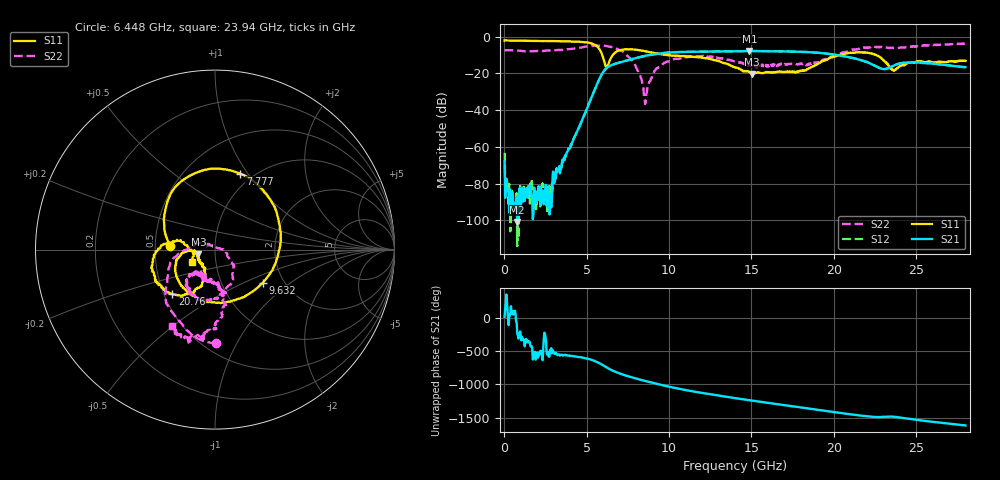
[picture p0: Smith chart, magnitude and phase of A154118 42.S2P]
!  2-Port S-parameters saved by WinCal
! VAR MeasName=S-Parameters (CALIBRATED_DATA) read from VNA (N5230A)
! VAR MeasDate=2015-9-10 14:37:42
! VAR NAME=A154118 42
! VAR FILENAME=A154118 42.S2P
! VAR DATE=2015-9-10 14:37:42
! VAR PHYS_PORTS=1,2
# Hz S DB R 50
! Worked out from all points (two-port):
!   801 points, 10 MHz to 28 GHz, reference 50 ohm
!   highest |S21| = -7.89 dB at 14.88 GHz (marker M1); lowest = -101.0 dB at 779.7 MHz (marker M2)
!   |S21| within 3 dB of the highest: 8.387 GHz to 20.75 GHz (12.37 GHz wide, 84.9 % of centre)
!   lowest |S11| = -20.3 dB at 15.05 GHz (marker M3), VSWR 1.21, Z = 41.5 - j2.24 ohm
!   |S11| at or under -10 dB: 5.938 GHz to 6.588 GHz (650.3 MHz wide, 10.4 % of centre); 9.806 GHz to 20.41 GHz (10.6 GHz wide, 70.2 % of centre); 22.58 GHz to end of sweep
!   |S22| runs from -36.7 to -3.7 dB; largest |S21 - S12| = 0.007
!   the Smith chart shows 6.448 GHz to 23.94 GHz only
!   S11 on the Smith chart (normalised r, x): 6.448 GHz: 0.60, +0.03; 7.777 GHz: 0.88, +0.92; 9.632 GHz: 1.57, -0.64; 20.76 GHz: 0.55, -0.31; 23.94 GHz: 0.76, -0.11
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1e7  -2.16 179.7  -67.96 19.1  -63.22 24.7  -7.49 179.8
1.849375e8  -2.16 177.2  -82.53 135.5  -82.31 15.3  -7.43 174.3
7.79725e8  -2.28 169.3  -100.98 121.6  -114.08 176.7  -7.60 155.9
2.774012e9  -2.49 142.1  -91.00 -118.1  -93.91 86.2  -7.66 97.4
4.698325e9  -3.00 98.2  -45.83 127.2  -45.63 127.0  -5.93 12.7
5.712962e9  -6.21 31.1  -24.14 47.7  -24.12 47.5  -4.94 -43.2
6.1678e9  -16.44 -82.5  -17.44 -17.7  -17.43 -17.8  -5.12 -71.3
6.4477e9  -11.97 175.2  -15.75 -56.6  -15.73 -57.0  -5.65 -89.4
7.777225e9  -7.02 71.4  -12.23 -175.4  -12.23 -175.5  -13.22 -170.3
8.54695e9  -7.97 30.1  -10.55 132.8  -10.53 132.9  -36.74 81.1
9.351662e9  -9.36 -17.8  -9.37 83.2  -9.31 83.0  -17.00 -43.3
9.631562e9  -9.79 -34.5  -9.04 67.1  -9.01 66.9  -14.90 -56.5
1.131096e10  -10.88 -118.1  -8.33 -17.7  -8.31 -18.4  -11.09 -95.9
1.4005e10  -16.74 -179.2  -8.02 -124.9  -8.02 -125.3  -13.55 -134.4
1.487969e10  -19.38 -168.9  -7.89 -156.6  -7.88 -157.3  -15.51 -127.0
1.505462e10  -20.33 -163.9  -7.91 -162.9  -7.91 -163.4  -15.25 -125.7
1.869332e10  -16.36 -110.6  -8.61 70.9  -8.61 70.3  -14.22 -90.2
2.075759e10  -9.26 -133.5  -10.89 -0.4  -10.88 -1.2  -8.34 -85.4
2.236701e10  -9.34 -175.1  -15.37 -47.3  -15.42 -47.9  -5.57 -106.5
2.334666e10  -16.08 171.3  -17.05 -42.7  -17.10 -43.5  -6.24 -117.7
2.394145e10  -16.61 -151.8  -14.80 -54.7  -14.77 -55.2  -6.22 -119.1
2.8e10  -13.26 -144.8  -16.66 -176.7  -16.74 -177.4  -3.68 -138.4
